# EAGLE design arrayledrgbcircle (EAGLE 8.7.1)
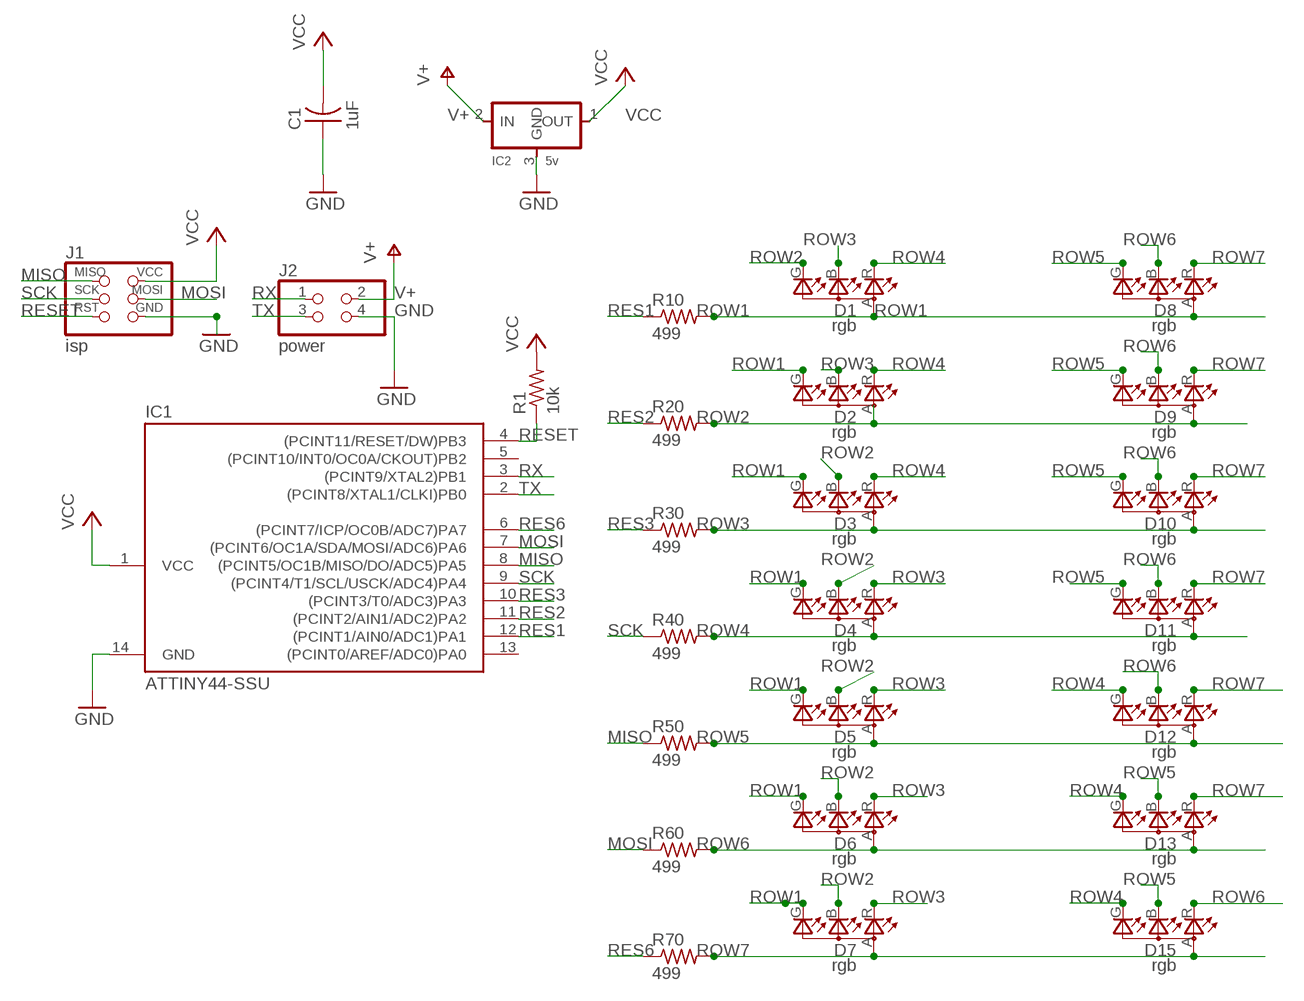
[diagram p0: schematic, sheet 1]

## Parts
C1  1uF  CAP-US1206FAB  [C1206FAB]
D1  rgb  LEDRGBNEW  [P-LCC-4]
D2  rgb  LEDRGBNEW  [P-LCC-4]
D3  rgb  LEDRGBNEW  [P-LCC-4]
D4  rgb  LEDRGBNEW  [P-LCC-4]
D5  rgb  LEDRGBNEW  [P-LCC-4]
D6  rgb  LEDRGBNEW  [P-LCC-4]
D7  rgb  LEDRGBNEW  [P-LCC-4]
D8  rgb  LEDRGBNEW  [P-LCC-4]
D9  rgb  LEDRGBNEW  [P-LCC-4]
D10  rgb  LEDRGBNEW  [P-LCC-4]
D11  rgb  LEDRGBNEW  [P-LCC-4]
D12  rgb  LEDRGBNEW  [P-LCC-4]
D13  rgb  LEDRGBNEW  [P-LCC-4]
D15  rgb  LEDRGBNEW  [P-LCC-4]
IC1  ATTINY44-SSU  [SOIC14]
IC2  5v  REGULATORSOT23  [SOT23]
J1  isp  AVRISPSMD  [2X03SMD]
J2  power  PINHD-2X2-SMD  [2X02SMD]
R1  10k  RES-US1206FAB  [R1206FAB]
R10  499  RES-US1206FAB  [R1206FAB]
R20  499  RES-US1206FAB  [R1206FAB]
R30  499  RES-US1206FAB  [R1206FAB]
R40  499  RES-US1206FAB  [R1206FAB]
R50  499  RES-US1206FAB  [R1206FAB]
R60  499  RES-US1206FAB  [R1206FAB]
R70  499  RES-US1206FAB  [R1206FAB]

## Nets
GND: C1.1 IC1.14(GND) IC2.3(GND) J1.6(GND) J2.4
MISO: IC1.8((PCINT5/OC1B/MISO/DO/ADC5)PA5) J1.1(MISO) R50.1
MOSI: IC1.7((PCINT6/OC1A/SDA/MOSI/ADC6)PA6) J1.4(MOSI) R60.1
RES1: IC1.12((PCINT1/AIN0/ADC1)PA1) R10.1
RES2: IC1.11((PCINT2/AIN1/ADC2)PA2) R20.1
RES3: IC1.10((PCINT3/T0/ADC3)PA3) R30.1
RES6: IC1.6((PCINT7/ICP/OC0B/ADC7)PA7) R70.1
RESET: IC1.4((PCINT11/RESET/DW)PB3) J1.5(RST) R1.1
ROW1: D1.A(A2) D2.G(CGREEN) D3.G(CGREEN) D4.G(CGREEN) D5.G(CGREEN) D6.G(CGREEN) D7.G(CGREEN) D8.A(A2) R10.2
ROW2: D1.G(CGREEN) D2.A(A2) D3.B(CBLUE) D4.B(CBLUE) D5.B(CBLUE) D6.B(CBLUE) D7.B(CBLUE) D9.A(A2) R20.2
ROW3: D1.B(CBLUE) D2.B(CBLUE) D3.A(A2) D4.R(CRED) D5.R(CRED) D6.R(CRED) D7.R(CRED) D10.A(A2) R30.2
ROW4: D1.R(CRED) D2.R(CRED) D3.R(CRED) D4.A(A2) D11.A(A2) D12.G(CGREEN) D13.G(CGREEN) D15.G(CGREEN) R40.2
ROW5: D5.A(A2) D8.G(CGREEN) D9.G(CGREEN) D10.G(CGREEN) D11.G(CGREEN) D12.A(A2) D13.B(CBLUE) D15.B(CBLUE) R50.2
ROW6: D6.A(A2) D8.B(CBLUE) D9.B(CBLUE) D10.B(CBLUE) D11.B(CBLUE) D12.B(CBLUE) D13.A(A2) D15.R(CRED) R60.2
ROW7: D7.A(A2) D8.R(CRED) D9.R(CRED) D10.R(CRED) D11.R(CRED) D12.R(CRED) D13.R(CRED) D15.A(A2) R70.2
RX: IC1.3((PCINT9/XTAL2)PB1) J2.1
SCK: IC1.9((PCINT4/T1/SCL/USCK/ADC4)PA4) J1.3(SCK) R40.1
TX: IC1.2((PCINT8/XTAL1/CLKI)PB0) J2.3
V+: IC2.2(IN) J2.2
VCC: C1.2 IC1.1(VCC) IC2.1(OUT) J1.2(VCC) R1.2
Unconnected: IC1.5((PCINT10/INT0/OC0A/CKOUT)PB2) IC1.13((PCINT0/AREF/ADC0)PA0)

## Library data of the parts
C1 = fab.lbr:CAP-US
D1-D13 D15 = fab.lbr:LEDRGBNEW
IC1 = fab.lbr:ATTINY44
IC2 = fab.lbr:REGULATOR
J1 = fab.lbr:AVRISP
J2 = fab.lbr:PINHD-2X2-SMD
R1 R10 R20 R30 R40 R50 R60 R70 = fab.lbr:RES-US: Resistor (US Symbol)

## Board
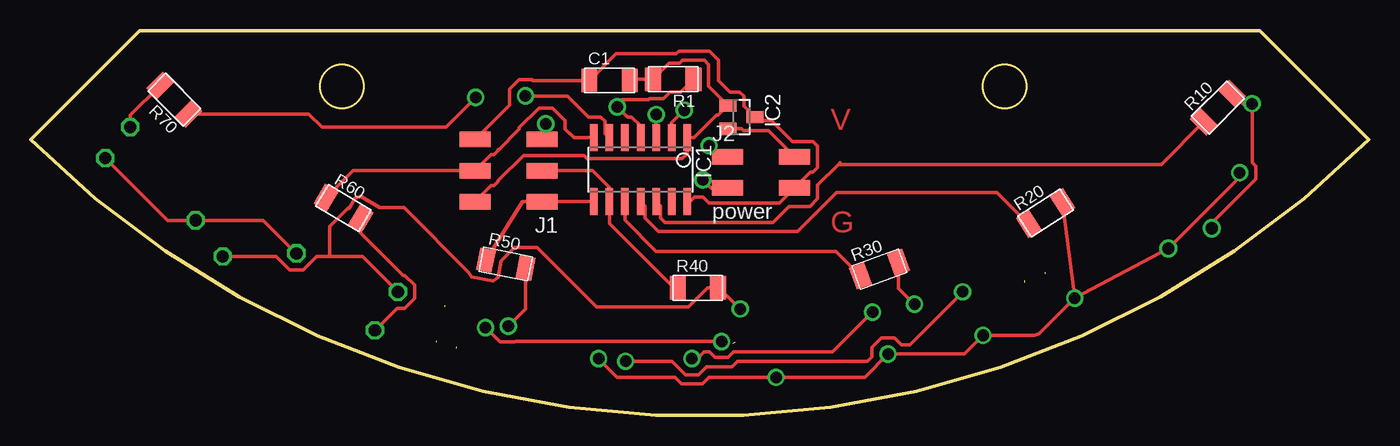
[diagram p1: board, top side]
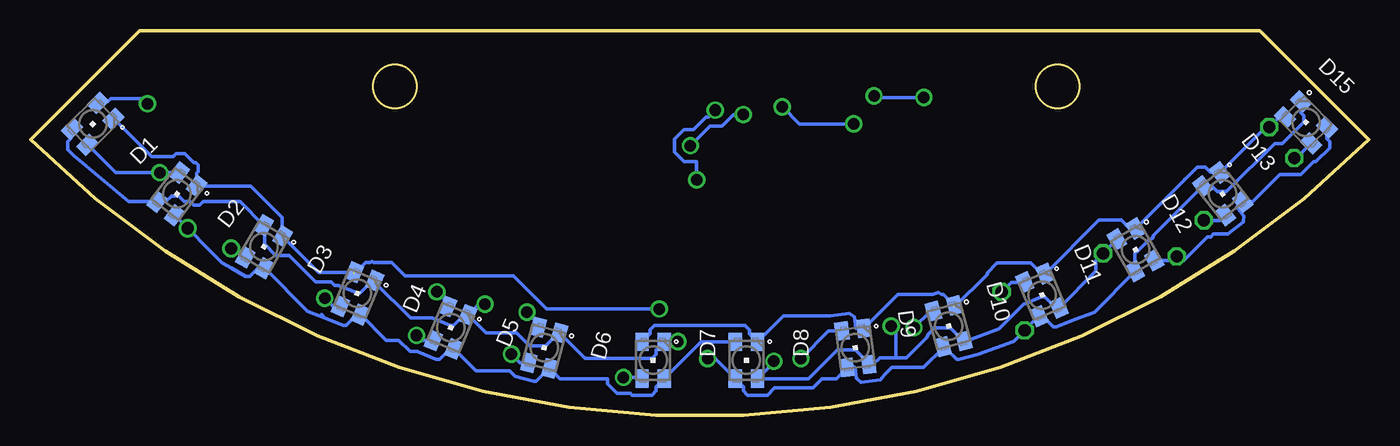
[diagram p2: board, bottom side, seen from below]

Size 109.22 x 31.43 mm. Coordinates in mm from the lower left corner, seen from the top.
Outline: 0,22.54 8.89,31.43 100.33,31.43 109.22,22.54 arc-90 0,22.54
Outline: circle at 25.4,26.86 radius 1.78
Outline: circle at 79.5,26.86 radius 1.78
Copper layers (1*16): Top 0.035mm / dielectric 1.5mm / Bottom 0.035mm
Design rules "basbasic *": minimum track width 0.3mm, minimum drill 0.9mm, track to track 0.45mm, track to pad 0.45mm, pad to pad 0.45mm, via to via 0.45mm, smd to smd 6mil, copper to edge 40mil, drill to drill 6mil, minimum pad ring 10mil, minimum via ring 8mil, stop-mask expansion 4mil, vias tented up to drill 0mil, thermal gap 10mil

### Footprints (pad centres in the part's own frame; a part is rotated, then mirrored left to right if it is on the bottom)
C1206FAB = smd 1.27 x 1.905: 1 -1.651,0; 2 1.651,0
P-LCC-4 = smd 1.1 x 1.5: A 0.902,-1.5; B 0.902,1.5; G -0.902,1.5; R -0.902,-1.5
SOIC14 = smd 0.61 x 2.21: 1 -3.81,-2.603; 2 -2.54,-2.603; 3 -1.27,-2.603; 4 0,-2.603; 5 1.27,-2.603; 6 2.54,-2.603; 7 3.81,-2.603; 8 3.81,2.603; 9 2.54,2.603; 10 1.27,2.603; 11 0,2.603; 12 -1.27,2.603; 13 -2.54,2.603; 14 -3.81,2.603
SOT23 = smd 1 x 1.4: 1 -0.95,-1.1; 2 0.95,-1.1; 3 0,1.1
2X03SMD = smd 2.54 x 1.27: 1 -2.54,2.54; 2 2.92,2.54; 3 -2.54,0; 4 2.92,0; 5 -2.54,-2.54; 6 2.92,-2.54
2X02SMD = smd 2.54 x 1.27: 1 -2.54,1.27; 2 2.92,1.27; 3 -2.54,-1.27; 4 2.92,-1.27
R1206FAB = smd 1.27 x 1.905: 1 -1.651,0; 2 1.651,0

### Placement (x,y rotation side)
C1  47.25,27.36 0 top
D1  104.14,23.81 135 bottom
D2  97.28,18.09 142.5 bottom
D3  90.17,13.77 150 bottom
D4  82.55,9.96 157.5 bottom
D5  74.93,7.17 157.5 bottom
D6  67.31,5.52 165 bottom
D7  58.42,4.5 180 bottom
D8  50.8,4.5 180 bottom
D9  41.91,5.52 187.5 bottom
D10  34.29,7.3 195 bottom
D11  26.67,9.84 202.5 bottom
D12  19.05,13.52 210 bottom
D13  11.94,18.09 218 bottom
D15  5.13,23.93 225 bottom
IC1  49.78,20.07 180 top
IC2  58.01,24.36 270 top
J1  39.21,19.99 180 top
J2  59.42,19.86 0 top
R1  52.45,27.45 180 top
R10  96.9,25.14 45 top
R20  82.83,16.53 32.5 top
R30  69.27,11.95 20 top
R40  54.45,10.42 0 top
R50  38.78,12.36 348.8 top
R60  25.53,16.94 329.1 top
R70  11.73,25.78 135 top

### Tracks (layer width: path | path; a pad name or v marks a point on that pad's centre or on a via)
GND
  Top 0.305: IC1.14 53.82,17.47 54.18,17.83 54.88,17.83 55.36,17.35 55.88,17.35 56.12,17.35 61.1,17.35 J2.4 63.64,19.89 63.86,19.89 64.21,20.24 64.21,22.01 63.86,22.36 62.17,22.36 60.45,24.08 59.39,24.08 IC2.3 58.22,25.25 58.22,26.06 57.86,26.41 57.06,26.41 56.13,27.34 56.13,29.01 55.39,29.76 52.9,29.76 52.66,29.52 47.77,29.52 C1.1 40.97,27.36 40.93,27.4 39.84,27.4 39.08,26.63 39.08,25.32 J1.6
MISO
  Top 0.305: IC1.8 45.95,17.45 J1.1 40.16,17.45 R50.1
MOSI
  Top 0.305: 38.16,21.65 37.81,21.29 37.59,21.29 J1.4 26.32,19.99 R60.1 | 38.16,21.65 38.16,21.7 | IC1.7 44.36,22.67 43.99,23.05 43.94,23.05 43.62,23.37 43.62,24.07 42.58,25.11 41.5,25.11 39.88,23.49 39.88,23.36 38.16,21.65
RES1
  Top 0.305: 66.04,20.63 65.91,20.51 | 65.91,20.51 64.21,18.8 64.21,17.7 63.59,17.08 61.9,17.08 60.58,15.76 51.76,15.76 51.41,16.11 51.41,17.1 IC1.12 | 65.91,20.51 92.27,20.51 R10.1
RES2
  Top 0.305: IC1.11 50.14,17.1 50.14,16.11 51.25,15 62.58,15 64.97,17.39 64.97,17.4 65.79,18.22 78.86,18.22 R20.1
RES3
  Top 0.305: IC1.10 48.51,15.94 51.05,13.39 65.71,13.39 R30.1
RES6  (via drill 0.94)
  Top 0.305: IC1.6 46.88,23.04 46.88,24.03 46.52,24.38 45.53,24.38 43.82,26.09 v40.39,26.09 | R70.1 22.7,24.62 23.78,23.54 33.9,23.54 v36.32,25.97
  Bottom 0.305: v36.32,25.97 40.26,25.97 v40.39,26.09
RESET  (via drill 0.94)
  Top 0.305: J1.5 42.04,22.82 v42.04,23.81 | 48.13,25.46 v47.88,25.2 | R1.1 53.03,26.38 52.17,26.38 51.66,25.88 50.51,25.88 50.44,25.8 48.26,25.8 47.88,25.42 v47.88,25.2 | v47.88,25.2 48.7,24.38 49.06,24.38 49.78,23.66 IC1.4
  Bottom 0.305: v47.88,25.2 46.48,23.81 v42.04,23.81
ROW1  (via drill 0.94, 0.99)
  Top 0.305: R10.2 98.92,25.46 v99.69,25.46 99.69,20.66 99.99,20.37 99.99,19.29 96.41,15.71 v96.41,15.28
  Bottom 0.305: D8.A 54.52,6 D7.G 58.17,2.35 58.17,2 58.52,1.65 60.12,1.65 60.27,1.8 61.37,1.8 62.14,2.57 62.14,3 65.99,3 66.64,3.65 | D6.G 66.64,3.65 | 66.64,3.65 67.1,3.65 67.96,2.79 68.15,2.79 69.69,3.2 70.14,3.65 72.88,3.65 D5.G 74.98,5.44 75.85,4.57 76.12,4.57 77.59,5.19 77.63,5.23 78.27,5.23 79.17,6.13 80.19,6.13 D4.G 82.6,8.23 83.47,7.37 83.74,7.37 85.21,7.98 | 85.21,7.98 85.47,8.23 | D1.A 102.92,25.63 102.68,25.88 100.12,25.88 v99.69,25.46 | 85.21,7.98 86.6,8.48 D3.G 90.66,12.02 91.33,11.36 91.68,11.36 92.84,12.02 93.57,12.44 D2.G v96.41,15.28
ROW2  (via drill 0.94, 0.99)
  Top 0.305: v46.36,4.63 47.88,3.11 52.58,3.11 53.12,2.57 54.83,2.57 55.37,3.11 v60.83,3.11 68.07,3.11 v69.98,5.01 76.2,5.01 v77.72,6.54 81.93,6.54 82.31,6.67 v85.22,9.58 | v98.68,19.83 98.68,19.46 | 98.68,19.46 98.68,19.24 | 98.68,19.46 v92.85,13.63 v85.22,9.58 | v85.22,9.58 R20.2
  Bottom 0.305: D1.G 102.28,19.83 v98.68,19.83 D2.A | D9.A 44.1,6.89 v46.36,4.63 | v60.83,3.11 59.43,3.11 D7.B | D5.B 77.32,6.13 v77.72,6.54 | v69.98,5.01 69.27,4.3 D6.B | v85.22,9.58 84.56,8.92 D4.B | 91.18,12.93 D3.B 92.42,13.52 92.96,13.52 v92.85,13.63
ROW3  (via drill 0.94)  (2 unrouted)
  Top 0.305: v56.39,6.03 39.57,6.03 39.53,5.99 38.31,5.99 v37.13,7.17 | v72.14,9.08 70.82,10.39 R30.2
  Bottom 0.305: D5.R 72.05,6.74 69.55,6.74 68.5,5.69 67.19,5.69 66.14,6.74 D6.R 63.97,4.65 58.52,4.65 58.17,5 58.17,5.35 D7.R | D5.R 73.83,8.21 74.7,7.35 74.97,7.35 76.44,7.96 78.22,7.96 81.14,10.88 81.45,10.88 82.32,10.01 82.59,10.01 84.06,10.62 84.41,10.62 84.68,10.89 85.97,10.89 88.14,13.05 89.21,13.05 90.14,13.98 90.14,15.33 D3.A 92.13,17.45 95.14,17.45 95.41,17.17 95.93,17.17 96.2,17.45 96.69,17.45 97.15,17.91 97.72,17.91 98.18,17.45 D2.B 101.23,17.45 105.72,21.22 106.21,21.71 106.21,22.34 105.96,22.59 D1.B | 57.92,5.87 57.33,5.87 57.18,6.03 v56.39,6.03 | D10.A 35.79,8.51 v37.13,7.17 | D5.R 72.66,9.08 v72.14,9.08
ROW4  (via drill 0.94, 0.99)  (1 unrouted)
  Top 0.305: v57.91,8.69 56.19,10.42 R40.2 55.24,10.42 53.68,8.86 46.19,8.86 41.32,13.73 39.51,13.73 38.41,12.63 38.14,11.26 37.73,10.98 35.99,11.32 35.76,11.67 30.46,16.97 28.5,16.97 26.98,17.88 26.5,17.75 25.98,16.88 25.91,16.95 24.38,15.43 24.38,12.99 | v29.97,10.09 27.08,12.99 24.38,12.99 | 24.38,12.99 23.34,12.99 22.25,11.89 21.13,11.89 20.04,12.99 v15.67,12.99
  Bottom 0.305: D1.R 99.35,21.14 97.58,21.14 97.32,21.39 96.66,21.39 95.91,20.63 95.76,20.63 95.56,20.44 95.56,19.89 95.65,19.8 D2.R 91.27,18.73 88.7,16.17 88.7,14.69 D3.R 85.71,11.7 D4.A | v57.91,8.69 67.11,8.69 69.82,11.4 78.65,11.4 79.76,12.5 81.23,12.5 81.36,12.56 81.5,12.5 81.87,12.5 82.81,11.57 | D12.G 15.75,12.67 | 15.75,12.67 15.1,12.67 13.18,14.59 12.9,14.59 12.7,14.8 11.52,14.8 10.26,15.78 10.2,16.28 10.77,17 D13.G 9.48,17.47 7.28,19.67 5.54,19.67 4.49,20.71 4.32,20.71 3.19,21.85 3.19,22.34 3.43,22.59 D15.G | D11.A 29.19,10.88 v29.97,10.09 | v15.67,12.99 15.67,12.74 15.75,12.67
ROW5  (via drill 0.94, 0.99)  (1 unrouted)
  Top 0.305: v38.99,7.3 40.4,8.71 R50.2 | v48.55,4.42 52.34,4.42 53.43,3.32 54.52,3.32 55.16,3.97 57.24,3.97 57.69,4.42 68.31,4.42 68.67,4.77 68.67,5.55 69.44,6.32 70.52,6.32 71.07,5.77 71.75,5.77 v76.07,10.09 | v6.1,21.01 11.18,15.93 v13.46,15.93 18.99,15.93 v21.69,13.24
  Bottom 0.305: 33.14,5.97 30.19,7.05 28.19,9.05 26.71,9.66 26.44,9.66 25.57,8.8 D11.G 22.26,11.8 22.26,12.66 v21.69,13.24 21.69,13.26 D12.A | 38.61,4.7 39.91,4.7 40.46,4.15 D9.G 41.27,4.6 41.27,4.76 41.3,4.76 41.9,5.36 43.36,5.36 43.56,5.15 43.58,5.15 45.73,3 D8.G 48.55,4.35 v48.55,4.42 | D10.G 33.12,6.08 34.17,7.13 35.48,7.13 35.82,6.79 35.82,6.73 35.9,6.71 36.11,6.34 37.75,4.7 38.61,4.7 | 38.61,4.7 38.61,6.92 v38.99,7.3 | v76.07,10.09 75.19,9.21 D5.A | D15.B 5.93,21.01 v6.1,21.01 | v13.46,15.93 12.15,15.93 D13.B
ROW6  (via drill 0.94, 0.99)  (1 unrouted)
  Top 0.305: v68.71,8.44 65.44,5.17 57.38,5.17 56.93,4.72 55.85,4.72 55.4,5.17 54.97,5.17 54.43,4.63 v53.98,4.63 | v28.1,6.95 29.89,8.75 30.53,8.75 31.32,9.53 31.32,10.65 30.53,11.44 30.41,11.44 26.95,14.9 R60.2
  Bottom 0.305: D11.B 26.62,8.11 25.75,7.24 25.48,7.24 24.01,7.85 22.42,8.43 D12.B 19.08,13.21 18.9,13.39 18.89,13.44 18.79,13.5 17.99,14.31 17.65,14.5 17.6,14.69 D13.A 12.83,18.72 12.38,18.27 11.63,18.27 7.7,22.21 7.07,22.21 5.31,23.97 5.31,24.47 5.55,24.71 D15.R | D9.B 42.55,3.91 | 42.55,3.91 41.95,3.91 41.83,3.01 41.44,2.7 39.85,2.91 39.55,3.31 38.94,3.91 36.35,3.91 34.77,5.49 34.55,5.49 33.64,4.57 33.45,4.57 31.91,4.98 28.99,6.04 D11.B | 42.55,3.91 43.46,3 44.63,3 45.38,2.25 48.5,2.25 49.1,1.65 50.7,1.65 51.05,2 51.05,2.35 D8.B 53.33,4.63 v53.98,4.63 | v68.71,8.44 67.79,7.53 D6.A | D11.B 26.94,8.11 v28.1,6.95
ROW7  (via drill 0.99)  (1 unrouted)
  Top 0.305: R70.2 8.13,24.51 v8.13,23.55
  Bottom 0.305: 33.9,8.85 33.81,8.85 31.15,11.51 31.15,11.65 30.37,12.43 27.59,12.43 26.72,11.57 D11.R 22.04,15.94 20.21,15.94 19.54,15.27 D12.R 15.04,19.25 15.03,19.29 14.86,19.43 14.01,20.28 13.34,20.28 12.96,19.89 12.09,19.89 | D7.A 58.67,6.65 58.67,7 58.32,7.36 50.9,7.36 50.55,7 50.55,6.65 D8.R 47.78,8.13 43.97,8.13 42.38,8.33 41.99,8.03 41.87,7.12 D9.R 38.44,9.9 35.6,9.9 35.13,10.03 34.91,9.9 34.73,9.9 D10.R | D15.A 7.32,24.36 v8.13,23.55 8.43,23.55 12.09,19.89 | D13.R 12.09,19.89
RX  (via drill 0.94)
  Top 0.305: J2.1 56.28,21.13 v55.37,22.03 | IC1.3 v51.05,24.56 v51.05,24.57
  Bottom 0.305: v55.37,22.03 53.78,23.63 52.8,23.63 51.85,24.57 v51.05,24.57
SCK
  Top 0.305: J1.3 45.85,19.99 47.24,18.6 47.24,18.59 IC1.9 47.24,15.68 52.51,10.42 R40.1
TX  (via drill 0.94)
  Top 0.305: IC1.2 52.32,23.91 v53.34,24.93 | v54.86,19.23 55.51,18.59 J2.3
  Bottom 0.305: v54.86,19.23 54.86,20.69 54.89,20.72 55.91,20.72 56.68,21.49 56.68,22.57 55.91,23.34 55.13,23.34 54.09,24.38 53.89,24.38 v53.34,24.93
V+
  Top 0.305: 56.88,23.37 IC2.2 58.01,23.41 58.16,23.25 60.21,23.25 J2.2
VCC
  Top 0.305: J1.2 37.59,18.75 37.81,18.75 38.16,19.11 38.16,19.16 40.23,21.23 45.15,21.23 45.41,20.97 53.16,20.97 53.59,21.39 53.59,21.4 IC1.1 54.13,22.67 55.96,24.51 56.12,24.51 IC2.1 55.34,26.88 55.34,28.66 54.98,29.01 53.22,29.01 52.98,28.77 52.11,28.77 R1.2 49,27.45 C1.2

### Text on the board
Top: V | G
